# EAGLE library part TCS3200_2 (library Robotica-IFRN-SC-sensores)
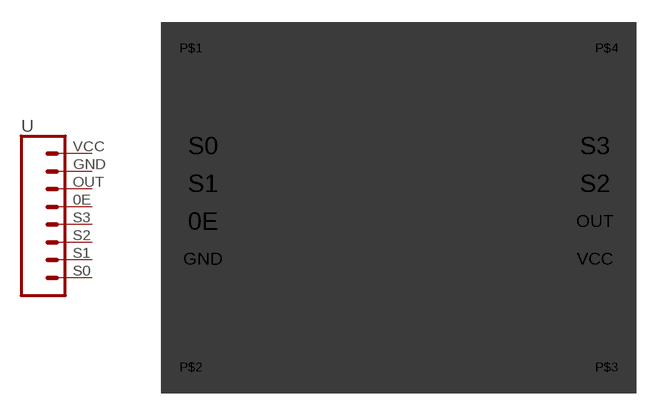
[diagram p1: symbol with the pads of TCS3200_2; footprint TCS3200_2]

Designator prefix -

## TCS3200_2TCS3200_2  [TCS3200_2]
0E  0E  pas
GND  GND  pas
OUT  OUT  pas
S0  S0  pas
S1  S1  pas
S2  S2  pas
S3  S3  pas
VCC  VCC  pas

## Footprint TCS3200_2 (pad centres in mm)
drill 1.118 pad 1.88 long: 0E -4.69,-2.67; GND -4.69,-5.21; OUT 21.71,-2.67; S0 -4.69,2.41; S1 -4.69,-0.13; S2 21.71,-0.13; S3 21.71,2.41; VCC 21.71,-5.21
drill 0.9: P$1 -5.5,9; P$2 -5.5,-12.5; P$3 22.5,-12.5; P$4 22.5,9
